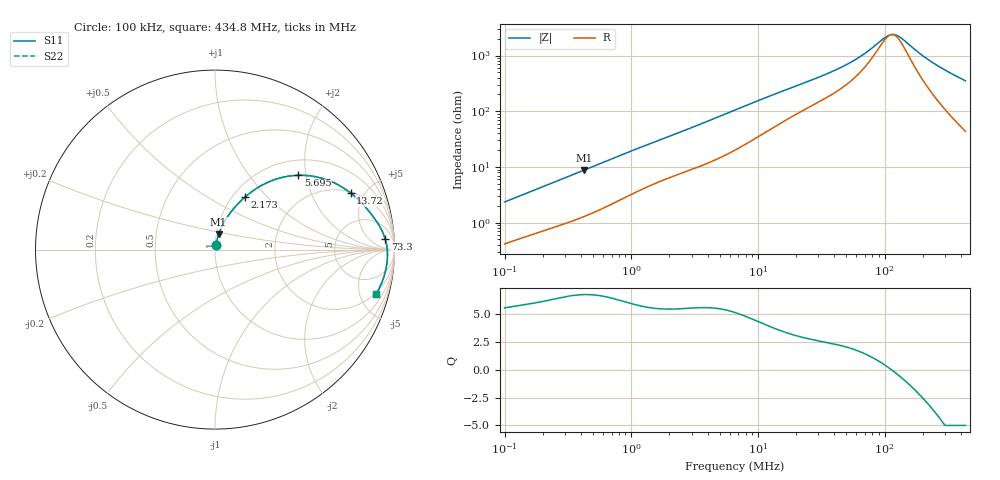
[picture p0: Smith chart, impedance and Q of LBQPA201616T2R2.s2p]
! LBQPA201616T2R2  S-PARAMETER MODEL  ( General Type )
! Model Generated by TAIYO YUDEN Corporation (http://www.ty-top.com)
! Version 1.0
! TAIYO YUDEN Control No. 191025NI43SB-FBB
! Copyright(c) 2019 TAIYO YUDEN CO.,LTD. All Rights Reserved.
! Product Description (link to TY-COMPAS)
! https://ds.yuden.co.jp/TYCOMPAS/or/detail?pn=LBQPA201616T2R2M&u=M
! Products Name : Inductors
! Characteristics :
!  Inductance : 2.2 uH , SRF(min) : 70 MHz , DC Resistance(max) : 0.26 Ohm
!  Rated Current : Saturation :750 mA , Temp Rise : 625 mA (20 degC)
!  Case Size : 2.0 x 1.6 / 0.079 x 0.063 [mm/inch] , Thickness : 1.6 / 0.063 [mm/inch]
!  (Conditions: Temperature = 25 degC , DC Bias Current/Voltage = 0A / 0V)
! External Node Assignments :
!  1  o---GGG---o  2
! GND o---------o GND
! Frequency Range : 0.1MHz  -  434.768421MHz  [ 402 STEP ]
# MHz S RI R 50
! Freq[MHz].  S11 Real  S11 Imag  S21 Real  S21 Imag  S12 Real  S12 Imag  S22 Real  S22 Imag
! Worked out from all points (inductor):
!   401 points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, 100 kHz to 434.8 MHz, reference 50 ohm
!   read as one part in series: L = 3.6 uH near 104.3 kHz
!   highest Q = 6.76 at 424.2 kHz (marker M1), where L = 3.27 uH
!   self-resonance near 113.6 MHz
!   S11 on the Smith chart (normalised r, x): 100 kHz: 1.01, +0.05; 2.173 MHz: 1.14, +0.75; 5.695 MHz: 1.34, +1.80; 13.72 MHz: 2.07, +3.96; 73.3 MHz: 15, +19; 434.8 MHz: 1.87, -6.98
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0.1  0.00467 0.0229  0.9953 -0.0229  0.9953 -0.0229  0.00467 0.0229
0.406826  0.019 0.0812  0.981 -0.0812  0.981 -0.0812  0.019 0.0812
0.424228  0.02 0.0843  0.98 -0.0843  0.98 -0.0843  0.02 0.0843
0.90166  0.0549 0.16  0.9451 -0.16  0.9451 -0.16  0.0549 0.16
1.65507  0.1208 0.2473  0.8792 -0.2473  0.8792 -0.2473  0.1208 0.2473
2.173  0.1673 0.2928  0.8327 -0.2928  0.8327 -0.2928  0.1673 0.2928
3.4448  0.2826 0.3696  0.7174 -0.3696  0.7174 -0.3696  0.2826 0.3696
5.694551  0.4637 0.414  0.5363 -0.414  0.5363 -0.414  0.4637 0.414
6.733248  0.5294 0.4109  0.4706 -0.4109  0.4706 -0.4109  0.5294 0.4109
9.816264  0.6642 0.3719  0.3358 -0.3719  0.3358 -0.3719  0.6642 0.3719
13.72387  0.7555 0.3154  0.2445 -0.3154  0.2445 -0.3154  0.7555 0.3154
26.82484  0.8666 0.2027  0.1334 -0.2027  0.1334 -0.2027  0.8666 0.2027
48.21867  0.9232 0.119  0.0768 -0.119  0.0768 -0.119  0.9232 0.119
73.30408  0.9477 0.0611  0.0523 -0.0611  0.0523 -0.0611  0.9477 0.0611
98.28046  0.9571 0.0204  0.0429 -0.0204  0.0429 -0.0204  0.9571 0.0204
109.1303  0.9591 0.00571  0.0409 -0.00571  0.0409 -0.00571  0.9591 0.00571
118.6665  0.9602 -0.00621  0.0398 0.00621  0.0398 0.00621  0.9602 -0.00621
129.0359  0.9608 -0.0183  0.0392 0.0183  0.0392 0.0183  0.9608 -0.0183
188.1188  0.9579 -0.0762  0.0421 0.0762  0.0421 0.0762  0.9579 -0.0762
231.9469  0.9516 -0.1122  0.0484 0.1122  0.0484 0.1122  0.9516 -0.1122
317.5582  0.9334 -0.1734  0.0666 0.1734  0.0666 0.1734  0.9334 -0.1734
434.7684  0.8993 -0.2449  0.1007 0.2449  0.1007 0.2449  0.8993 -0.2449
